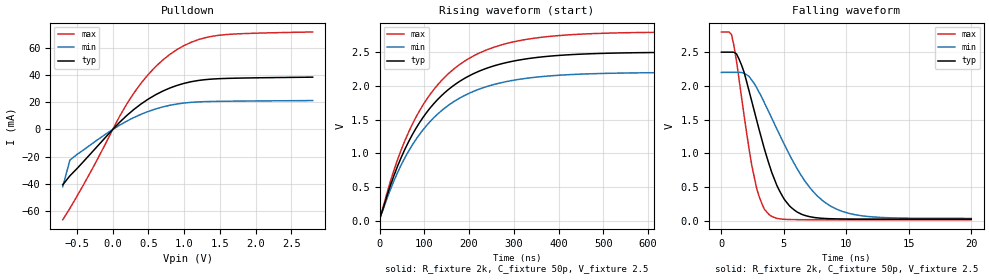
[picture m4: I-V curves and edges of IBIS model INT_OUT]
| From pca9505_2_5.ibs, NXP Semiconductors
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[Model]   INT_OUT
Model_type Open_drain
Vref=2.5
Vmeas=1.25
Rref=2k
Cref=50p
C_comp   5.2p   5p   5.4p
[Temperature Range] 27   85   -40
[Voltage Range]   2.5   2.2   2.8
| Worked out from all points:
|   slope of the pulldown table from 0 to 0.375 V, typ, clamps not added: 21.1 ohm
|   falling waveform, R_fixture 2k, C_fixture 50p, V_fixture 2.5: 20-80 % time 2.35ns typ, 3.79ns min, 1.41ns max; typ from 2.5 V to 0.022 V
|   rising waveform, R_fixture 2k, C_fixture 50p, V_fixture 2.5: 20-80 % time 141ns typ, 142ns min, 141ns max; typ from 0.022 V to 2.5 V
[Pulldown]
-700mV    -40.51mA   -41.9mA    -66.09mA
-600mV    -33.94mA   -22.43mA   -57.78mA
-500mV    -28.63mA   -18.29mA   -48.81mA
-200mV    -11.46mA   -7.098mA   -20.4mA
100mV     5.434mA    3.245mA    9.958mA
300mV     14.82mA    8.837mA    26.97mA
500mV     22.32mA    13.24mA    40.43mA
800mV     30.35mA    17.7mA     54.98mA
1.1V      34.99mA    19.87mA    63.89mA
1.4V      36.94mA    20.52mA    68.32mA
1.8V      37.64mA    20.78mA    70.14mA
2.8V      38.3mA     21.15mA    71.4mA
[Falling Waveform]
R_fixture=2k
C_fixture=50p
V_fixture=2.5
V_fixture_min=2.2
V_fixture_max=2.8
0s        2.5V       2.2V       2.8V
808.1ps   2.5V       2.2V       2.762V
1.616ns   2.307V     2.199V     1.827V
2.424ns   1.776V     2.087V     825mV
3.03ns    1.343V     1.902V     353mV
3.838ns   824.5mV    1.596V     85.29mV
5.657ns   183.8mV    904.6mV    14.99mV
7.273ns   51.08mV    446.1mV    13.49mV
8.889ns   26.9mV     200.7mV    13.45mV
20ns      22.07mV    32.59mV    13.45mV
[Rising Waveform]
R_fixture=2k
C_fixture=50p
V_fixture=2.5
V_fixture_min=2.2
V_fixture_max=2.8
0s        22.07mV    32.46mV    13.45mV
40.4ns    811.4mV    715.7mV    908.6mV
64.65ns   1.168V     1.029V     1.309V
88.89ns   1.45V      1.276V     1.626V
113.1ns   1.672V     1.471V     1.875V
145.5ns   1.897V     1.669V     2.127V
210.1ns   2.181V     1.918V     2.444V
282.8ns   2.344V     2.062V     2.626V
387.9ns   2.444V     2.151V     2.738V
800ns     2.499V     2.199V     2.799V
[Ramp]
R_load=2k
dV/dt_r   1.487E+0/2.821E-9   1.478E+0/3.129E-9   1.493E+0/2.474E-9
dV/dt_f   1.487E+0/2.220E-10   1.478E+0/3.458E-10   1.493E+0/1.169E-10
|[End   INT_OUT
